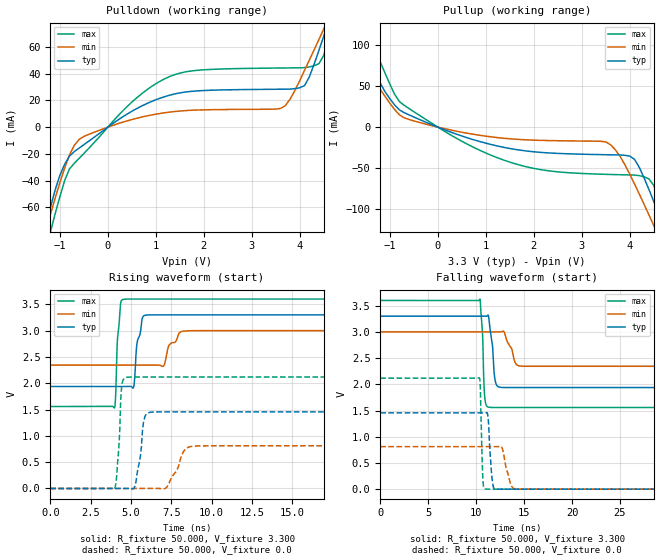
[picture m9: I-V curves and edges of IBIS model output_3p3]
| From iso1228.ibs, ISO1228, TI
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|   Model output_3p3
[Model] output_3p3
Model_type Output
Polarity   Non-Inverting
Enable   Active-High
Vmeas = 1.65
Vref = 0
Cref = 15pF
Rref = 1000
C_comp   0.978pF   1.050pF   0.889pF
[Temperature Range]   27.000   0.150k   -40.000
[Voltage Range]   3.300V   3.000V   3.600V
[Pullup Reference]   3.300V   3.000V   3.600V
[Pulldown Reference]   0.0V   0.0V   0.0V
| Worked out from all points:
|   slope of the pulldown table from 0 to 0.495 V, typ, clamps not added: 42.2 ohm
|   slope of the pullup table from 0 to 0.495 V, typ, clamps not added: 46.1 ohm
|   rising waveform, R_fixture 50.000, V_fixture 3.300: 20-80 % time 356ps typ, 721ps min, 207ps max; typ from 1.94 V to 3.3 V
|   rising waveform, R_fixture 50.000, V_fixture 0.0: 20-80 % time 353ps typ, 726ps min, 213ps max; typ from 0 V to 1.46 V
|   falling waveform, R_fixture 50.000, V_fixture 3.300: 20-80 % time 410ps typ, 815ps min, 246ps max; typ from 3.3 V to 1.94 V
|   falling waveform, R_fixture 50.000, V_fixture 0.0: 20-80 % time 294ps typ, 603ps min, 184ps max; typ from 1.46 V to 0 V
[Pulldown]
|Voltage   I(typ)   I(min)   I(max)
-3.3V     -447.8mA   -372.8mA   -654.4mA
-1.3V     -74.39mA   -77.85mA   -94.82mA
-1.2V     -60.33mA   -65.41mA   -78.6mA
-900mV    -27.72mA   -30.46mA   -39.85mA
-600mV    -15.68mA   -9.201mA   -23.38mA
500mV     11.84mA    5.676mA    18.66mA
1.3V      23.95mA    11.27mA    37.96mA
3.6V      28.3mA     13.97mA    44.16mA
4.1V      31.01mA    42.51mA    44.42mA
4.5V      67.87mA    73.32mA    53.59mA
4.7V      89mA       89.09mA    81.73mA
6.6V      358.2mA    289.3mA    493.9mA
[Pullup]
|Voltage   I(typ)   I(min)   I(max)
-3.3V     356.7mA    258.7mA    567mA
-2.1V     161.1mA    122.4mA    246.9mA
-1.8V     121.5mA    96.5mA     180.5mA
-1.5V     87.45mA    71.23mA    126mA
-700mV    17.66mA    11.4mA     26.61mA
1.4V      -24.96mA   -13.72mA   -40.75mA
3.5V      -33.67mA   -18.07mA   -57.65mA
4.1V      -39.42mA   -69.47mA   -58.55mA
4.4V      -76.17mA   -107.2mA   -63.21mA
4.6V      -105.6mA   -132.9mA   -86.69mA
4.8V      -135.9mA   -159mA     -125.7mA
6.6V      -482.2mA   -443.3mA   -617.5mA
[Ramp]
| variable   typ   min   max
dV/dt_r   0.873/0.354n   0.487/0.726n   1.271/0.213n
dV/dt_f   0.817/0.414n   0.394/0.817n   1.225/0.244n
R_load = 50.000
[Rising Waveform]
R_fixture= 50.000
V_fixture= 3.300
V_fixture_min= 3.000
V_fixture_max= 3.600
|time   V(typ)   V(min)   V(max)
0s        1.938V     2.344V     1.558V
3.98ns    1.938V     2.344V     1.531V
4.16ns    1.938V     2.344V     2.804V
4.36ns    1.938V     2.344V     3.516V
4.67ns    1.938V     2.344V     3.599V
5.18ns    1.941V     2.344V     3.6V
5.4ns     2.794V     2.344V     3.6V
6.06ns    3.299V     2.344V     3.6V
8.67ns    3.3V       2.998V     3.6V
100ns     3.3V       3V         3.6V
[Rising Waveform]
R_fixture= 50.000
V_fixture= 0.0
V_fixture_min= 0.0
V_fixture_max= 0.0
|time   V(typ)   V(min)   V(max)
0s        278.2nV    99.06nV    1.22nV
3.99ns    304.7nV    99.06nV    -6.058mV
4.25ns    295.6nV    99.06nV    775.1mV
4.43ns    426.1nV    99.06nV    1.949V
4.75ns    -36.4uV    99.06nV    2.114V
5.25ns    46.93mV    99.08nV    2.118V
5.81ns    1.306V     512.7nV    2.118V
6.34ns    1.453V     -29.93uV   2.118V
9.17ns    1.455V     809.3mV    2.118V
100ns     1.455V     810.9mV    2.118V
[Falling Waveform]
R_fixture= 50.000
V_fixture= 3.300
V_fixture_min= 3.000
V_fixture_max= 3.600
|time   V(typ)   V(min)   V(max)
0s        3.3V       3V         3.6V
10.4ns    3.3V       3V         3.625V
10.68ns   3.3V       3V         2.898V
10.77ns   3.3V       3V         2.213V
10.91ns   3.3V       3V         1.721V
11.41ns   3.112V     3V         1.561V
11.94ns   2.113V     3V         1.558V
12.52ns   1.943V     2.999V     1.558V
14.84ns   1.938V     2.345V     1.558V
100ns     1.938V     2.344V     1.558V
[Falling Waveform]
R_fixture= 50.000
V_fixture= 0.0
V_fixture_min= 0.0
V_fixture_max= 0.0
|time   V(typ)   V(min)   V(max)
0s        1.455V     810.9mV    2.118V
10.34ns   1.455V     810.9mV    2.121V
10.43ns   1.455V     810.9mV    1.952V
10.7ns    1.455V     810.9mV    194.1mV
10.99ns   1.455V     810.9mV    2.061mV
11.25ns   1.355V     810.9mV    383uV
11.75ns   79.15mV    810.9mV    99.23uV
12.27ns   587.8uV    810.4mV    27.59uV
14.35ns   9.877uV    1.214mV    478.1nV
100ns     28.18nV    118.3nV    9.148nV
